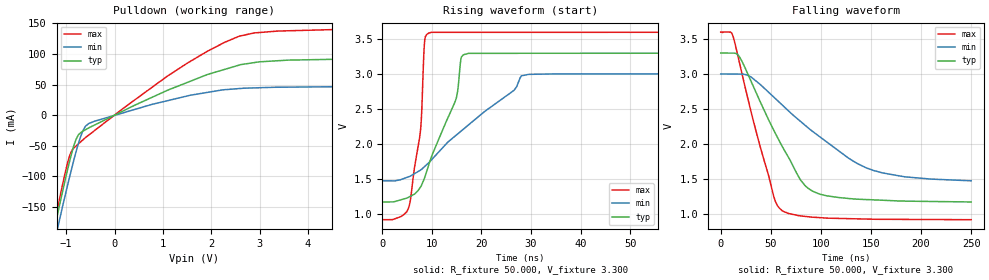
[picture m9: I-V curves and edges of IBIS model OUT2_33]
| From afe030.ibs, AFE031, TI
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|   OUT2 3.3V Model
[Model]  OUT2_33
Model_type   Open_drain
Polarity   Non-Inverting
Enable   Active-Low
Vmeas = 1.65
Vref = 1.65
Cref = 15pF
Rref = 50
|   typ   min   max
|   (nom PVT)   (slow PVT)   (fast PVT)
|   C_comp high output
C_comp   4.6970950e-12  3.5975860e-12  7.4857130e-12
|   typ   min   max
|   (nom PVT)   (fast PVT)   (slow PVT)
|   C_comp low output
|C_comp   2.1723070e-12  1.7879310e-12  2.5707980e-12
| Where   nom PVT is  Nominal Process, 3.3V, 52C
|   Fast PVT is Strong Process, 3.6V, -40C
|   Slow PVT is Weak Process, 3.0V, 150C
[Voltage Range]   3.3   3   3.6
[Temperature Range]   52   150   -40
[Pullup Reference]   3.3   3   3.6
[Pulldown Reference]   0   0   0
[Power Clamp Reference]   3.3   3   3.6
[GND Clamp Reference]   0   0   0
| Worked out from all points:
|   slope of the pulldown table from 0 to 0.495 V, typ, clamps not added: 26 ohm
|   falling waveform, R_fixture 50.000, V_fixture 3.300: 20-80 % time 44.3ns typ, 78.5ns min, 29.1ns max; typ from 3.3 V to 1.17 V
|   rising waveform, R_fixture 50.000, V_fixture 3.300: 20-80 % time 6.49ns typ, 15.2ns min, 2.13ns max; typ from 1.17 V to 3.3 V
[Pulldown]
|   Voltage   I(typ)   I(min)   I(max)
-3.3V     -1.005A    -982.8mA   -1.079A
-1.265V   -193.5mA   -215.6mA   -187.1mA
-1.124V   -142.1mA   -166.4mA   -131.6mA
-923mV    -73.48mA   -98.95mA   -64.9mA
-845.7mV  -50.85mA   -74.52mA   -54.11mA
-751.1mV  -32.75mA   -47.6mA    -47.36mA
-655.4mV  -26.21mA   -25.79mA   -40.53mA
-531.9mV  -20.91mA   -13.72mA   -32.57mA
1.101V    40.79mA    23.69mA    64.12mA
2.568V    81.54mA    43.32mA    128.6mA
3.381V    88.92mA    45.55mA    137.4mA
6.6V      94.19mA    47.84mA    144.1mA
[Ramp]
R_load = 50
|   typ   min   max
dV/dt_r   1.28076/6.48364e-009  0.902489/1.5118e-008   1.61281/2.13383e-009
dV/dt_f   1.28066/4.42973e-008  0.902261/7.84911e-008   1.6128/2.91397e-008
[Falling Waveform]
R_fixture = 50.000
V_fixture = 3.300
V_fixture_min = 3.000
V_fixture_max = 3.600
C_fixture = 0.000
|  time   V(typ)   V(min)   V(max)
0s        3.3V       3V         3.6V
12.03ns   3.299V     2.999V     3.551V
21.04ns   3.186V     2.998V     3.017V
30.49ns   2.889V     2.955V     2.447V
52.65ns   2.202V     2.673V     1.26V
61.65ns   1.955V     2.552V     1.037V
79.99ns   1.475V     2.316V     966.1mV
98.8ns    1.278V     2.101V     941.4mV
152.5ns   1.196V     1.617V     918.5mV
250ns     1.166V     1.469V     912mV
[Rising Waveform]
R_fixture = 50.000
V_fixture = 3.300
V_fixture_min = 3.000
V_fixture_max = 3.600
C_fixture = 0.000
|  time   V(typ)   V(min)   V(max)
0s        1.165V     1.469V     912mV
5.434ns   1.239V     1.53V      1.114V
7.735ns   1.384V     1.624V     2.219V
8.565ns   1.52V      1.675V     3.495V
9.874ns   1.805V     1.766V     3.595V
14.9ns    2.647V     2.122V     3.595V
15.95ns   3.243V     2.185V     3.595V
17.39ns   3.294V     2.27V      3.595V
29.54ns   3.295V     2.993V     3.595V
250ns     3.3V       3V         3.6V
